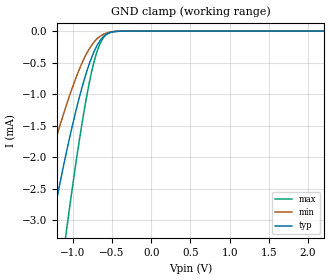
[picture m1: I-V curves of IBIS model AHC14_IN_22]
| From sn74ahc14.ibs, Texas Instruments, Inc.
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[Model]   AHC14_IN_22
Model_type  Input
Vinl=0.7
Vinh=1.43
| variable   typ   min   max
C_comp   0.57pF   0.52pF   0.63pF
[Temperature Range]   40   100   -40
| Ambient temperature   25   85   -40
[Voltage range]   2.2   2   2.4
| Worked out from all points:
|   GND clamp passes 1 mA (typ) near -0.91 V on its own axis
[GND Clamp]
| AHC14_IN_22
|   Voltage   I(typ)   I(min)   I(max)
-2.2V     -10.47mA   -6.806mA   -15.33mA
-1.545V   -5.032mA   -3.224mA   -7.897mA
-1.515V   -4.808mA   -3.077mA   -7.572mA
-1.29V    -3.218mA   -2.03mA    -5.205mA
-1.08V    -1.91mA    -1.165mA   -3.151mA
-945mV    -1.185mA   -691.5uA   -1.958mA
-820mV    -629.2uA   -346uA     -1.01mA
-720mV    -299.7uA   -159.7uA   -441.1uA
-625mV    -106.8uA   -60.34uA   -133.4uA
-545mV    -32.77uA   -20.84uA   -33.42uA
-420mV    -3.434uA   -2.379uA   -2.224uA
2.2V      1.234nA    466.5pA    2.192nA
